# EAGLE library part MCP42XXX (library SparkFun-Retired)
SPI controlled dual digital potentiometer by Microchip Not in catalog?
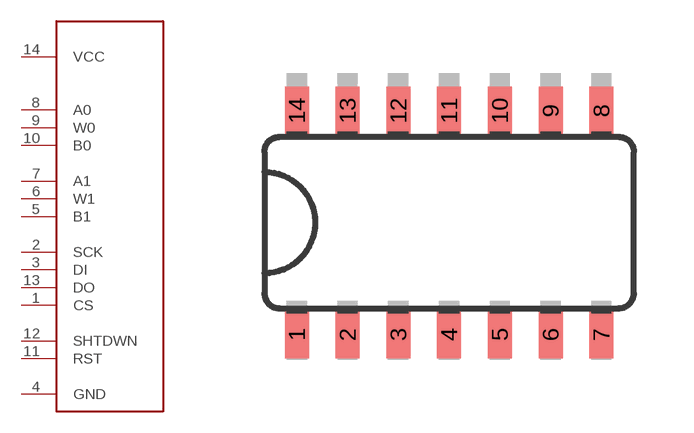
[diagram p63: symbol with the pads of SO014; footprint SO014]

Designator prefix U

## MCP42XXX  [SO014]
1  CS
2  SCK
3  DI
4  GND
5  B1
6  W1
7  A1
8  A0
9  W0
10  B0
11  RST
12  SHTDWN
13  DO
14  VCC

## Footprint SO014 (pad centres in mm)
smd 0.6 x 1.2: 1 -3.175,-2.8; 2 -1.905,-2.8; 3 -0.635,-2.8; 4 0.635,-2.8; 5 1.905,-2.8; 6 3.175,-2.8; 7 4.445,-2.8; 8 4.445,2.8; 9 3.175,2.8; 10 1.905,2.8; 11 0.635,2.8; 12 -0.635,2.8; 13 -1.905,2.8; 14 -3.175,2.8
